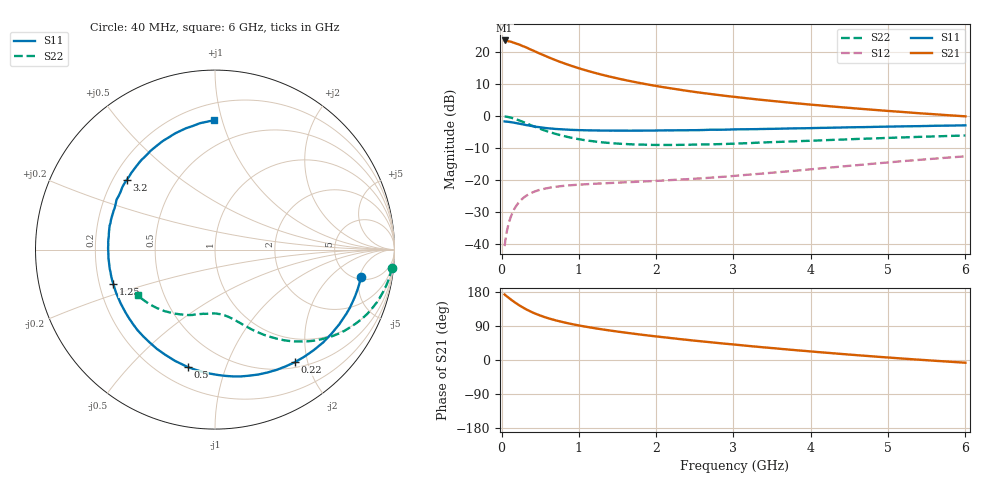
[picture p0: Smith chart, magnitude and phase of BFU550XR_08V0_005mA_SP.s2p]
! Filename:  P:\Prog\Test\Noise\ATS_data\Testdata_Net\03 Spar\BFU550XR_APG2013_45_C05_08p0V_005mA_SP_CM01_D.s2p
! Date/Time: Tue 06/Aug/2013 14:38:17
! BFU550XR_APG2013_45_C05_08p0V_1to35mA_SP_CM01_Bias4_R.s2p
! MDIF S-parameter v. bias file
! BFU550XR_APG2013_45_C05_08p0V_1to35mA_SP_CM01
! Date/time Fri Aug 02 14:53:20 2013
! VAR V_out= 8.0010
! VAR I_out= 4.9950
! VAR V_in= 0.8067
! VAR I_in= 0.0528
! Device data file deembeded for feedlines and parallel
! Original file: \03 Spar\BFU550XR_APG2013_45_C05_08p0V_005mA_SP_CM01_R.s2p
! Feed-files: PR006V01_02082013_Feed1.s2p, PR006V01_02082013_Feed2.s2p
! Parallel-file: PR006V01_02082013_Par.s2p
# MHz S MA R 50
!  Freq-MHz  S11-mag  S11-arg  S21-mag  S21-arg  S12-mag  S12-arg  S22-mag  S22-arg
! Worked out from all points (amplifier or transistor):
!   98 points, 40 MHz to 6 GHz, reference 50 ohm
!   highest |S21| = 23.7 dB at 40 MHz (marker M1)
!   |S21| within 3 dB of that: start of sweep to 393.5 MHz
!   unconditionally stable (mu >= 1): 2.41 GHz to 4.225 GHz
!   at 300 MHz: K = 0.17, MSG = 23.4 dB, |S12| = -25.2 dB
!   at 1.6 GHz: K = 0.77, MSG = 16.0 dB, |S12| = -20.7 dB
!   at 6 GHz: K = 0.84, MSG = 6.3 dB, |S12| = -12.5 dB
!   S11 on the Smith chart (normalised r, x): 40 MHz: 5.49, -5.29; 220 MHz: 0.58, -1.79; 500 MHz: 0.31, -0.75; 1.25 GHz: 0.26, -0.15; 3.2 GHz: 0.26, +0.33; 6 GHz: 0.31, +0.94
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40  0.8287 -10.5  15.26 172.9  0.009331 84.2  0.9902 -5.8
50  0.8266 -13.1  15.24 170.7  0.01152 83.1  0.9872 -7.4
120  0.8076 -31.1  14.61 159.8  0.02676 73.4  0.9514 -17.6
180  0.7853 -45.4  13.79 151.0  0.03805 66.1  0.9035 -25.4
220  0.7693 -54.6  13.31 145.6  0.04446 62.1  0.8677 -30.0
260  0.753 -62.8  12.68 140.6  0.05016 58.1  0.8317 -34.3
320  0.7274 -75.0  11.87 133.6  0.05719 53.1  0.7762 -40.0
420  0.6924 -91.7  10.46 123.9  0.06601 46.5  0.693 -47.6
500  0.6716 -103.0  9.464 117.5  0.07108 42.4  0.6368 -52.5
600  0.6482 -115.3  8.417 110.5  0.0755 38.5  0.5761 -57.6
750  0.6272 -129.7  7.117 102.2  0.08038 34.7  0.5105 -63.3
900  0.6129 -141.4  6.147 95.2  0.08359 32.2  0.4623 -67.8
1050  0.6048 -150.7  5.384 89.3  0.08589 30.8  0.4276 -71.7
1250  0.5983 -161.2  4.609 82.5  0.08875 29.8  0.3973 -75.9
1650  0.5946 -177.4  3.566 71.0  0.0933 29.9  0.3655 -83.3
2050  0.5992 170.1  2.899 61.1  0.09829 31.6  0.3559 -90.0
2500  0.6048 157.8  2.396 51.0  0.1057 33.9  0.3602 -97.1
3100  0.6252 143.7  1.953 39.0  0.1195 37.4  0.3761 -106.1
3200  0.6264 141.4  1.892 37.0  0.1222 37.8  0.3797 -107.6
4100  0.6565 123.4  1.482 20.9  0.1521 39.4  0.4182 -121.3
5200  0.695 103.5  1.162 3.6  0.1992 36.4  0.4668 -137.6
6000  0.7206 90.5  0.9957 -7.2  0.2361 31.6  0.5002 -149.3
